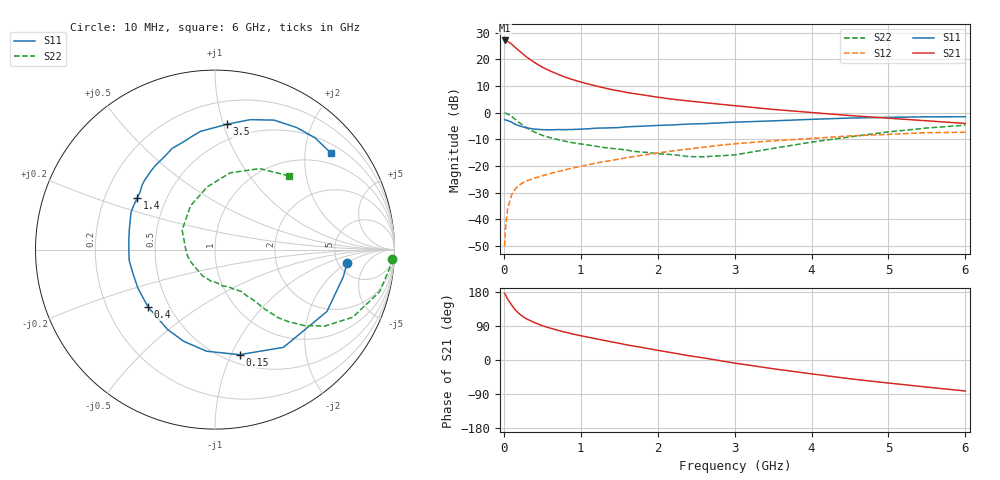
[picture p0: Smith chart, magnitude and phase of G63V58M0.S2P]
! SIEMENS Small Signal Semiconductors
! BFG193
! Si NPN RF Bipolar Junction Transistor in SOT223
! VCE = 3.5 V  IC = 8 mA
! Common Emitter S-Parameters:  August  1996
# GHz  S  MA  R  50
!  f  S11  S21  S12  S22
! GHz  MAG  ANG  MAG  ANG  MAG  ANG  MAG  ANG
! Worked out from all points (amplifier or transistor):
!   36 points, 10 MHz to 6 GHz, reference 50 ohm
!   highest |S21| = 27.2 dB at 10 MHz (marker M1)
!   |S21| within 3 dB of that: start of sweep to 163.6 MHz
!   unconditionally stable (mu >= 1): 945 MHz to 2.603 GHz
!   at 250 MHz: K = 0.47, MSG = 24.1 dB, |S12| = -26.3 dB
!   at 1.4 GHz: K = 1.08, MAG = 11.6 dB, |S12| = -17.9 dB
!   at 6 GHz: K = 0.88, MSG = 1.7 dB, |S12| = -7.4 dB
!   S11 on the Smith chart (normalised r, x): 10 MHz: 5.96, -2.03; 150 MHz: 0.59, -1.08; 400 MHz: 0.38, -0.32; 1.4 GHz: 0.34, +0.27; 3.5 GHz: 0.37, +1.03; 6 GHz: 0.71, +2.61
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0.01  0.7392 -6.0  22.79 175.7  0.0031 91.4  0.9875 -2.9
0.02  0.7308 -11.9  22.57 172.7  0.0064 84.6  0.9798 -5.9
0.05  0.7128 -28.9  21.83 160.3  0.0158 76.3  0.9463 -14.4
0.1  0.6648 -55.0  19.55 145.5  0.0282 66.6  0.8545 -26.2
0.15  0.6014 -76.8  16.76 131.5  0.0373 57.0  0.745 -34.9
0.2  0.5681 -94.7  14.57 122.2  0.0434 53.0  0.6552 -40.3
0.25  0.5401 -108.8  12.61 114.1  0.0485 49.5  0.5746 -44.4
0.3  0.5175 -120.7  11.01 108.0  0.0525 48.1  0.5191 -47.1
0.4  0.4913 -139.3  8.76 98.6  0.0588 46.5  0.4314 -50.1
0.5  0.4804 -153.2  7.162 90.5  0.0653 46.4  0.3754 -51.8
0.6  0.4761 -163.7  6.1 84.3  0.0718 46.6  0.3402 -53.4
0.7  0.482 -172.9  5.299 78.5  0.0779 46.9  0.3131 -55.4
0.9  0.4839 172.7  4.167 68.5  0.0918 46.8  0.2721 -58.3
1.1  0.4988 161.4  3.446 60.0  0.1053 46.4  0.2459 -64.3
1.4  0.5198 146.6  2.72 47.9  0.1267 44.3  0.2134 -73.7
1.7  0.5505 135.4  2.273 36.4  0.1507 41.3  0.1868 -85.6
2.2  0.5895 118.4  1.786 18.6  0.1917 33.4  0.1628 -114.6
2.8  0.6426 101.7  1.448 -1.4  0.2436 22.5  0.1546 -159.7
3.5  0.7019 84.5  1.153 -23.0  0.2963 6.7  0.2134 149.1
4.5  0.7928 65.5  0.884 -49.5  0.366 -13.2  0.3517 97.1
5.5  0.8359 48.0  0.704 -71.5  0.4217 -37.9  0.5155 61.1
6  0.8407 39.6  0.628 -81.8  0.4286 -52.1  0.5826 44.8
